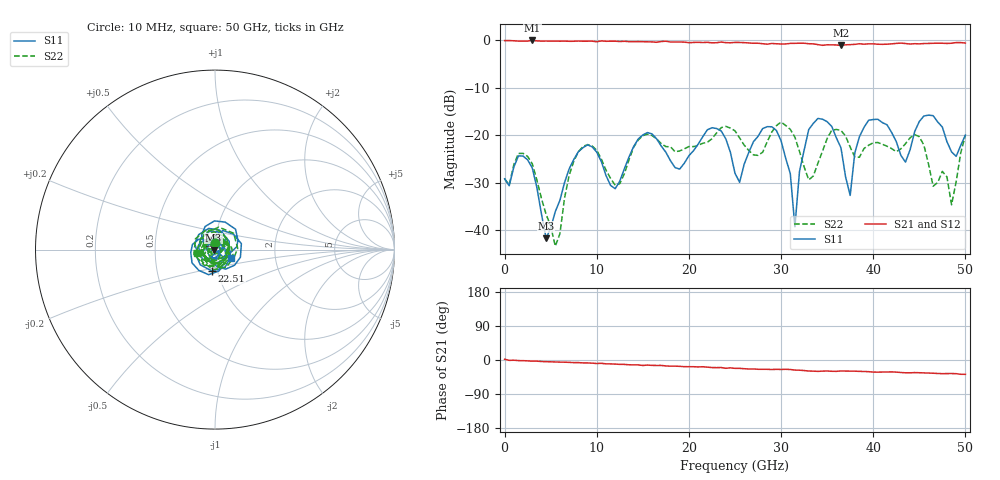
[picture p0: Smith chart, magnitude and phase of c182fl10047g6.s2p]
! 8/5/2019 3:04:47 PM
! Z:\MATT MILLER ENGINEERING\C182FL10047G6.S2P
! CHANNEL.1
! TR.MEASUREMENT
! CORRECTED.DATA
# GHZ S RI R 50.0
! FREQ.GHZ  S11RE  S11IM  S21RE  S21IM  S12RE  S12IM  S22RE  S22IM
!; PortSelection: Port_12
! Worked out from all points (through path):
!   101 points, 10 MHz to 50 GHz, reference 50 ohm
!   highest |S21| = 0.01 dB at 3.009 GHz (marker M1); lowest = -1.0 dB at 36.5 GHz (marker M2)
!   group delay of S21, straight-line fit = 2.07 ps
!   lowest |S11| = -41.7 dB at 4.509 GHz (marker M3), VSWR 1.02, Z = 49.2 - j0.271 ohm
!   |S11| at or under -10 dB: start of sweep to end of sweep
!   |S22| runs from -43.4 to -17.2 dB; largest |S21 - S12| = 0.027
!   S11 on the Smith chart (normalised r, x): 10 MHz: 0.99, +0.07; 22.51 GHz: 0.94, -0.23; 50 GHz: 1.19, -0.12
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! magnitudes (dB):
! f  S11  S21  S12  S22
! 10 MHz  -29.2  0.0  0.0  -29.2
! 3.009 GHz  -26.9  0.0  0.0  -26.0
! 4.509 GHz  -41.7  -0.1  -0.1  -36.6
! 5.509 GHz  -36.1  -0.1  -0.1  -43.4
! 8.508 GHz  -22.6  -0.2  -0.2  -22.3
! 12.01 GHz  -31.3  -0.1  -0.2  -30.5
! 17.01 GHz  -22.3  -0.2  -0.1  -21.8
! 19.01 GHz  -27.1  -0.3  -0.3  -23.3
! 22.51 GHz  -18.4  -0.5  -0.5  -20.7
! 25 GHz  -28.0  -0.4  -0.4  -19.0
! 29.5 GHz  -19.0  -0.7  -0.9  -17.9
! 31.5 GHz  -39.3  -0.6  -0.6  -20.4
! 32 GHz  -27.6  -0.6  -0.6  -23.4
! 33.5 GHz  -17.5  -0.7  -0.8  -28.6
! 36.5 GHz  -22.6  -1.0  -1.0  -19.0
! 37.5 GHz  -32.7  -0.9  -0.8  -22.5
! 39.5 GHz  -16.8  -0.7  -0.7  -22.1
! 42 GHz  -19.4  -0.7  -0.7  -22.8
! 43.5 GHz  -25.6  -0.6  -0.7  -21.8
! 45 GHz  -17.1  -0.7  -0.8  -20.3
! 48.5 GHz  -23.5  -0.6  -0.6  -34.7
! 50 GHz  -20.0  -0.5  -0.5  -20.0
